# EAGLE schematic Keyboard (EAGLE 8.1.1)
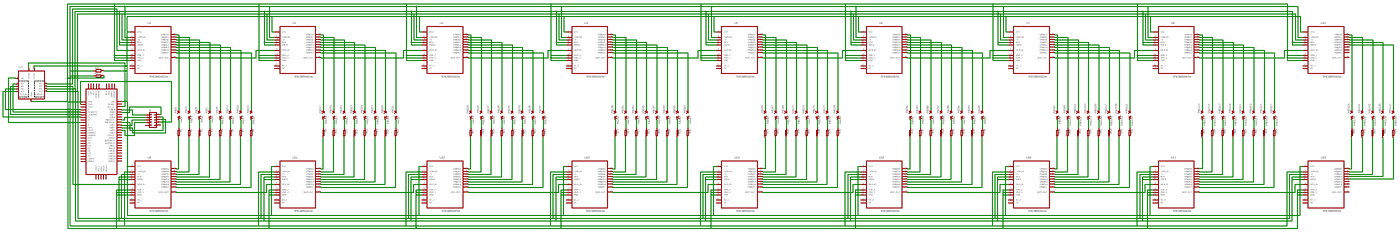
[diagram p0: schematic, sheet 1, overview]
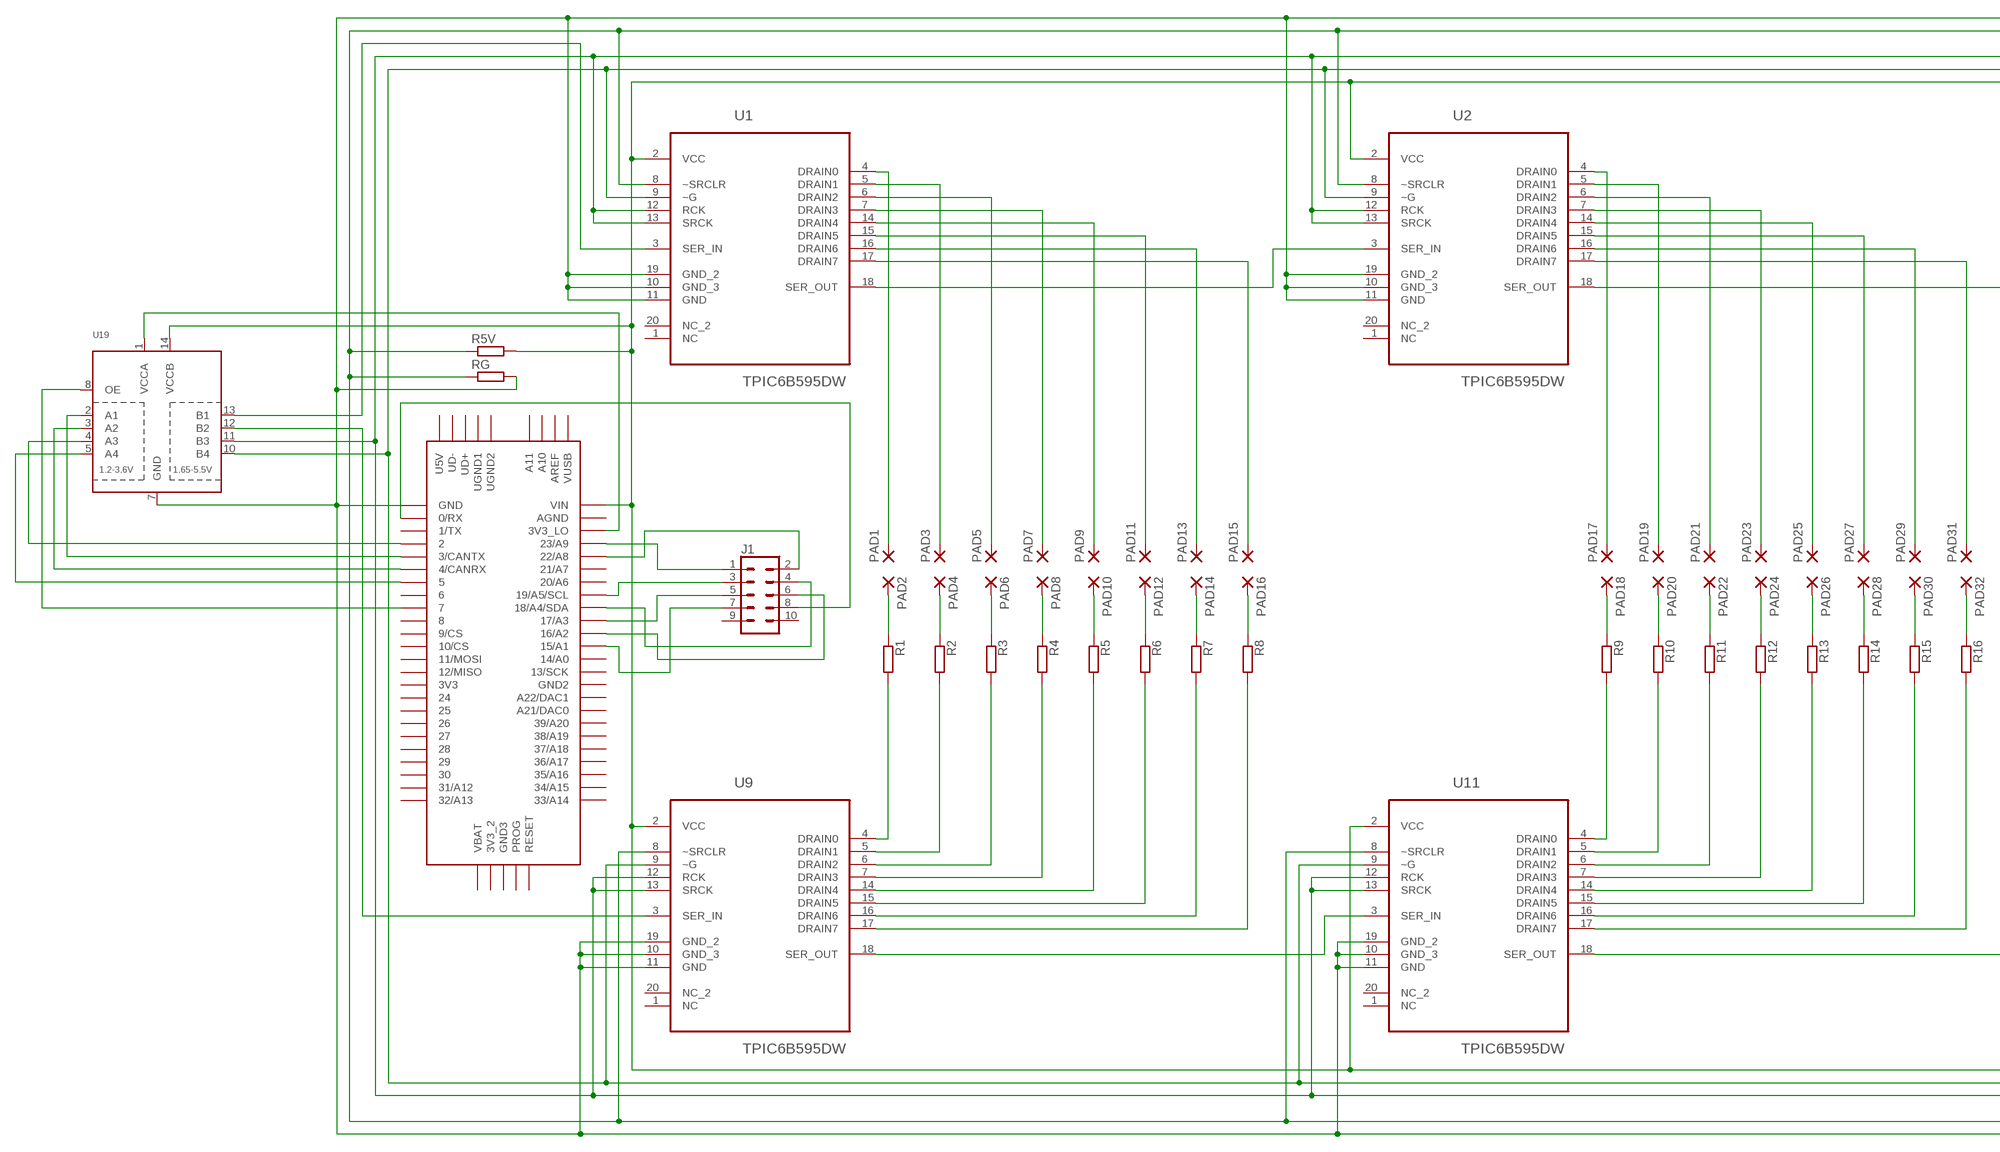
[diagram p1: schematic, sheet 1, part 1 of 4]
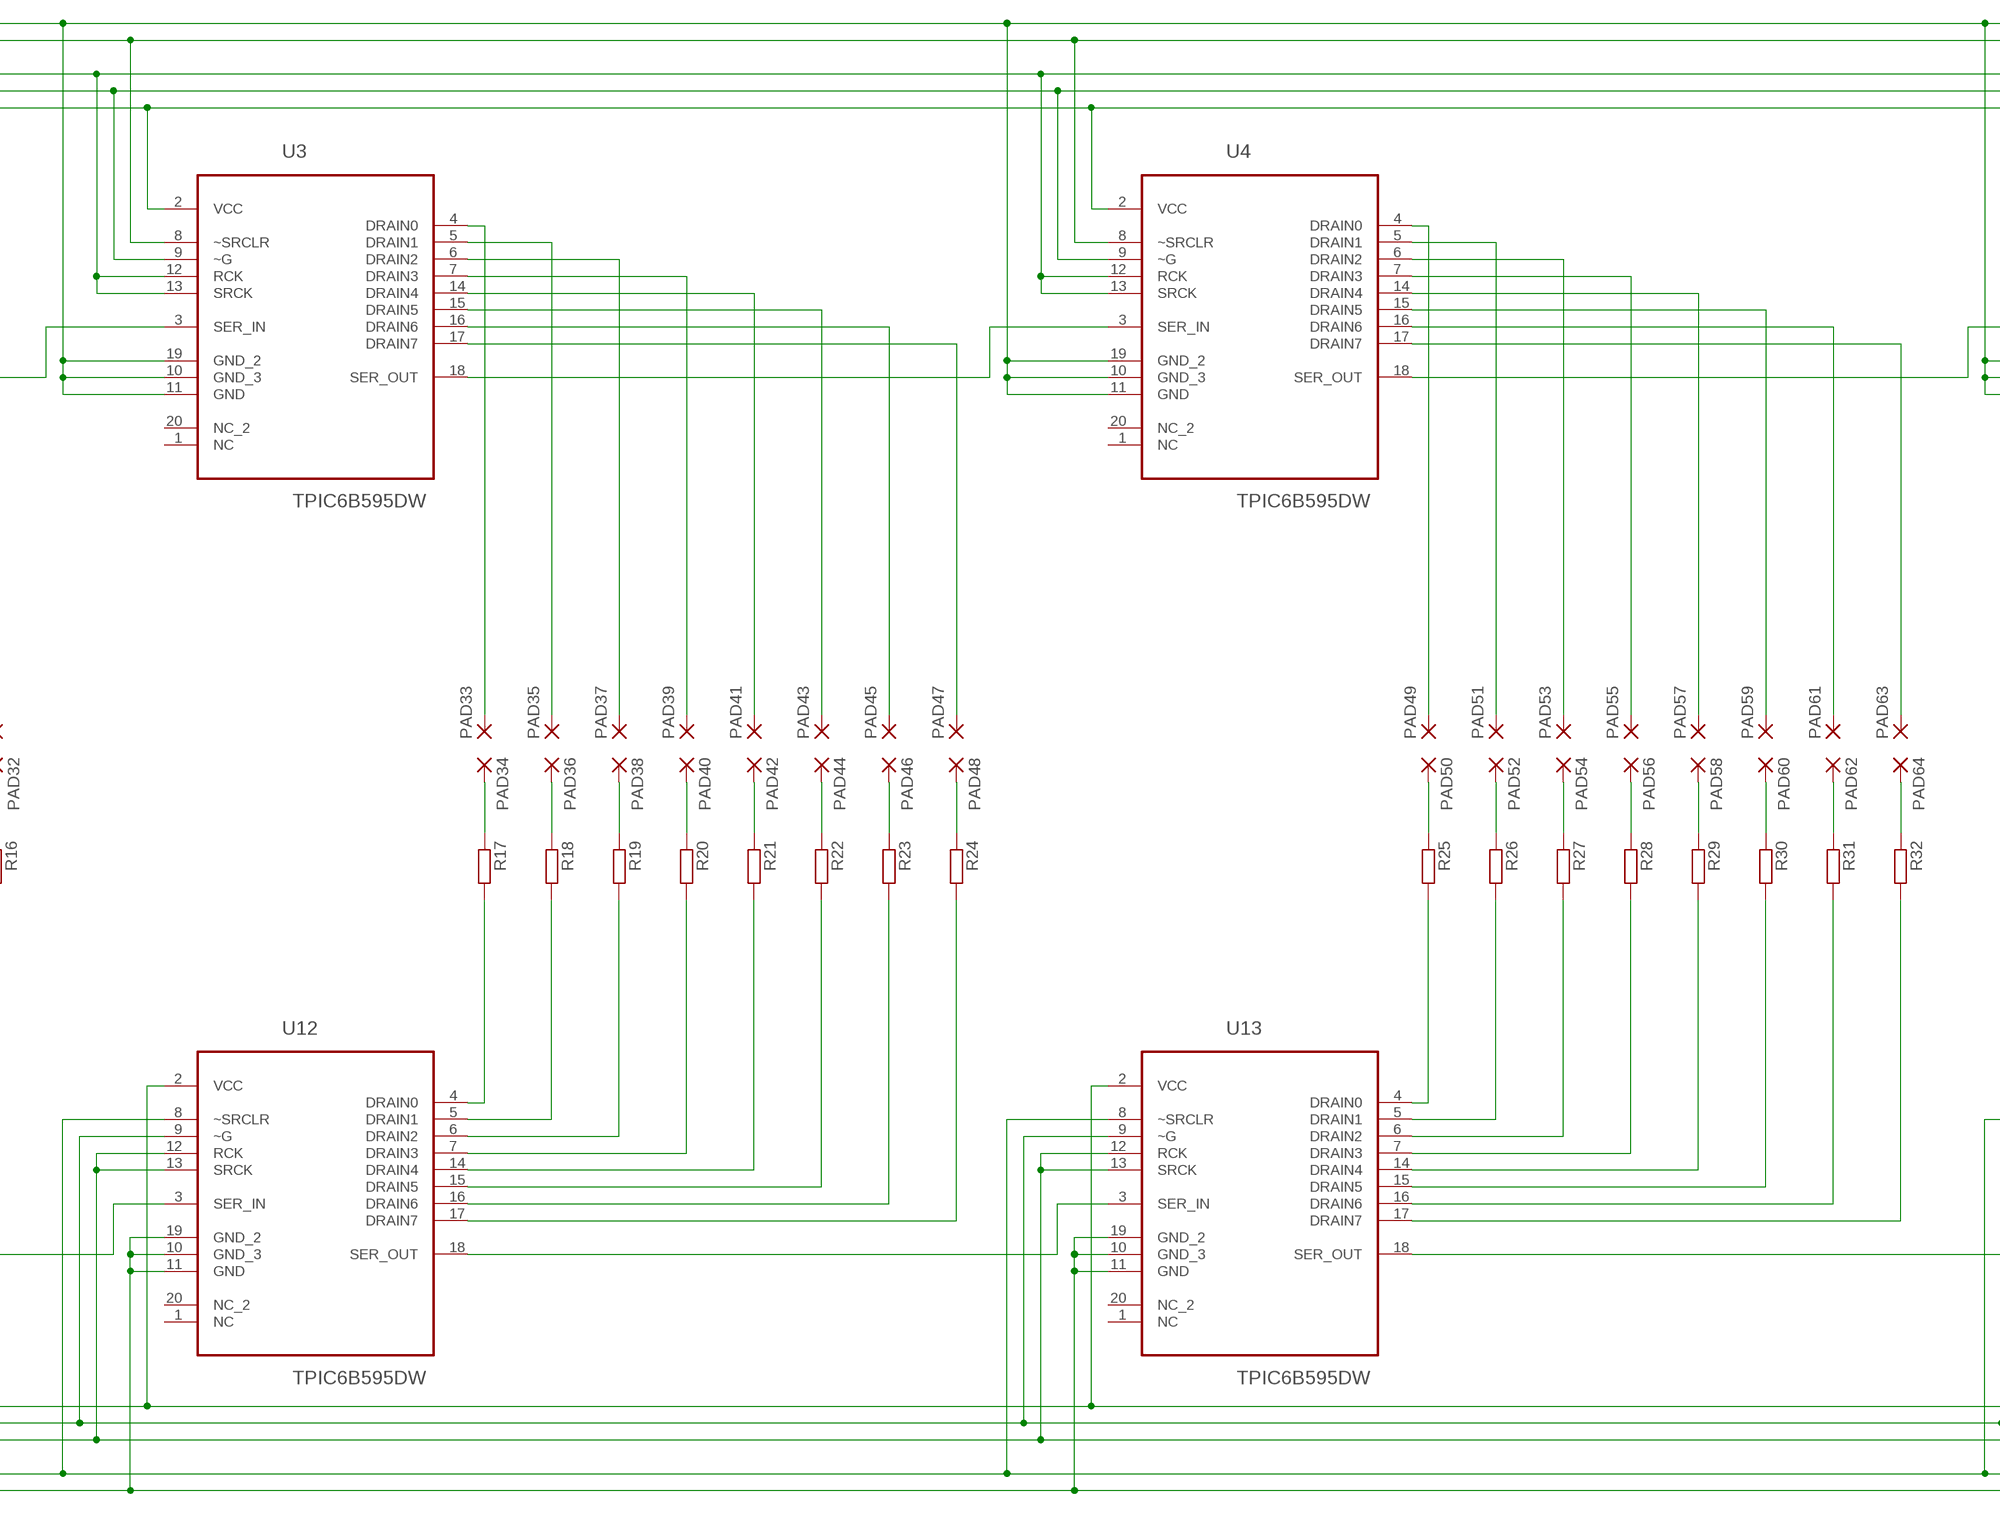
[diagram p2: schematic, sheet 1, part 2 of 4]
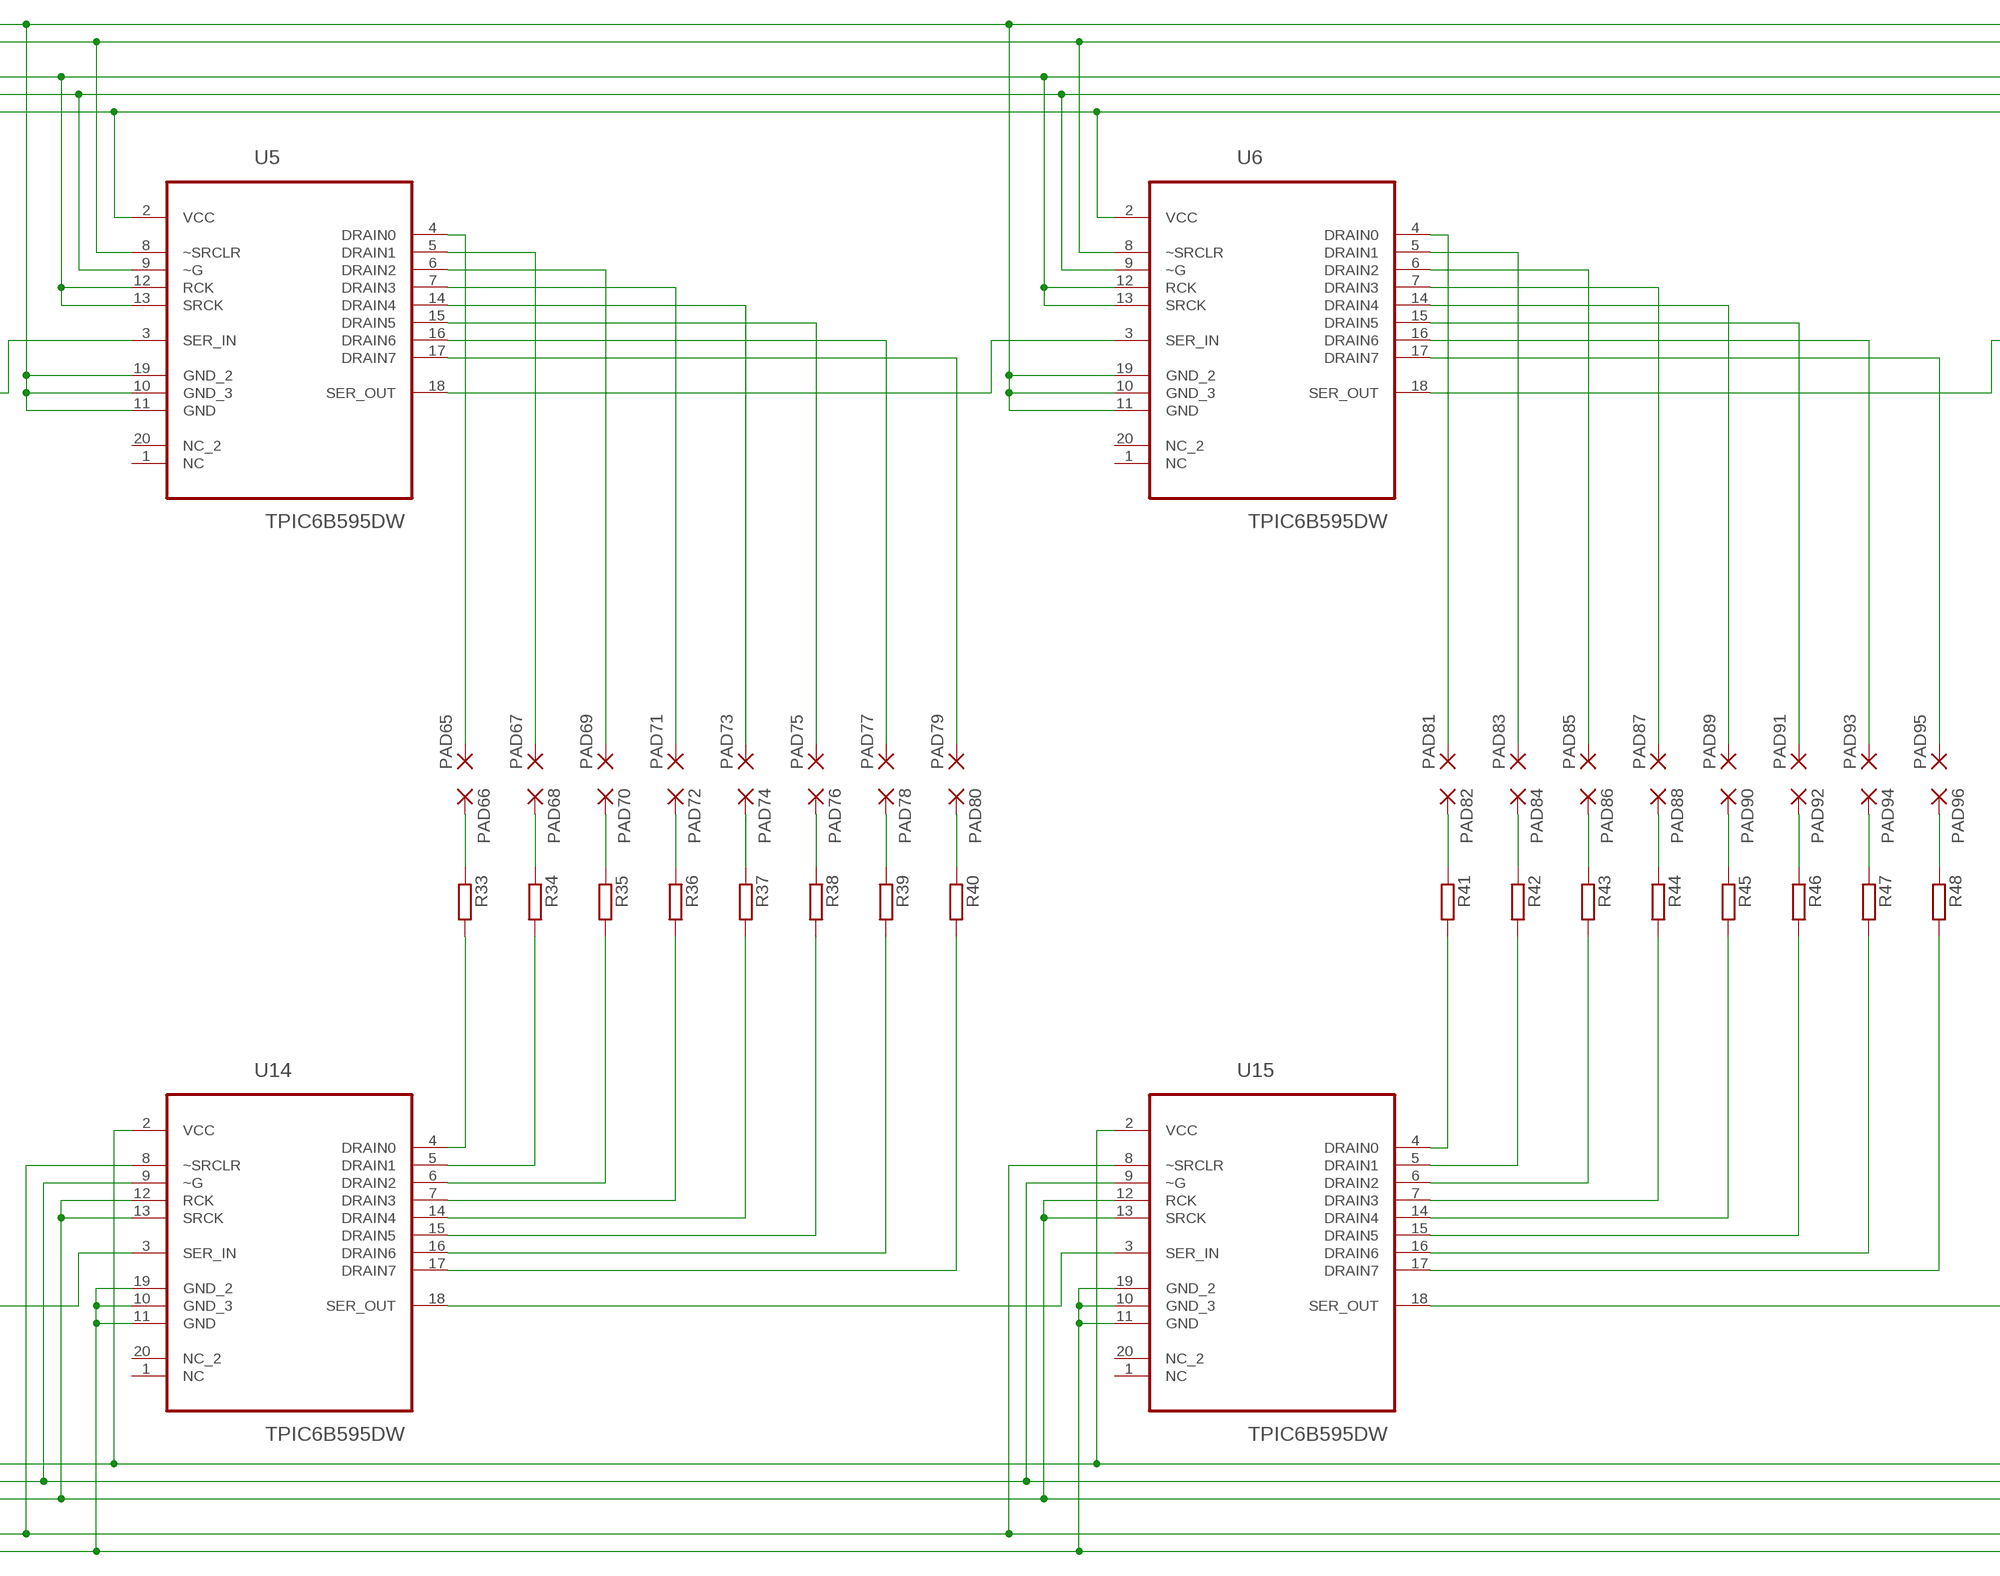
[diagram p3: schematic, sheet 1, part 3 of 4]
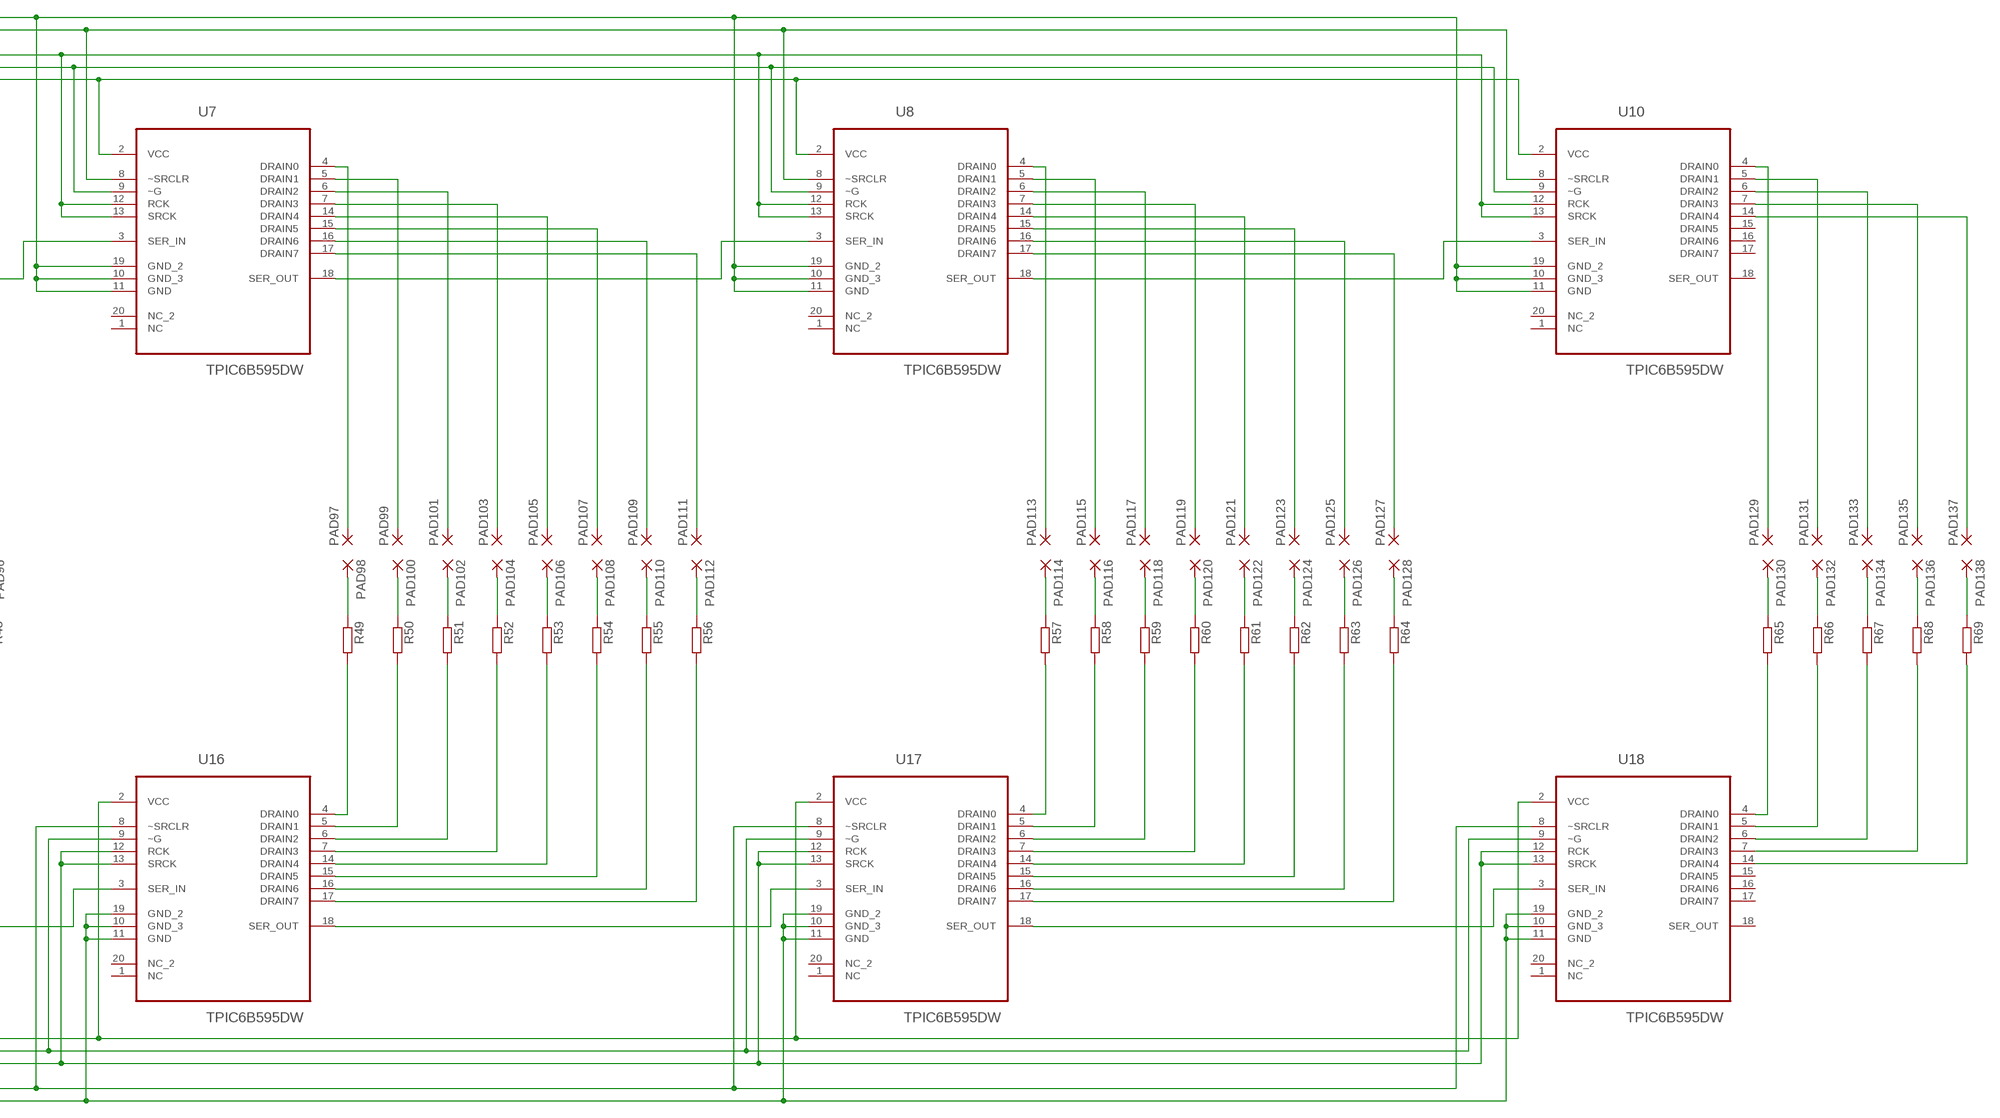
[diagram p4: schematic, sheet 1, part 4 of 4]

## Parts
J1  CONN_05X2SHD  [2X5-SHROUDED]
PAD1  1,6/0,8  [1,6/0,8]
PAD2  1,6/0,8  [1,6/0,8]
PAD3  1,6/0,8  [1,6/0,8]
PAD4  1,6/0,8  [1,6/0,8]
PAD5  1,6/0,8  [1,6/0,8]
PAD6  1,6/0,8  [1,6/0,8]
PAD7  1,6/0,8  [1,6/0,8]
PAD8  1,6/0,8  [1,6/0,8]
PAD9  1,6/0,8  [1,6/0,8]
PAD10  1,6/0,8  [1,6/0,8]
PAD11  1,6/0,8  [1,6/0,8]
PAD12  1,6/0,8  [1,6/0,8]
PAD13  1,6/0,8  [1,6/0,8]
PAD14  1,6/0,8  [1,6/0,8]
PAD15  1,6/0,8  [1,6/0,8]
PAD16  1,6/0,8  [1,6/0,8]
PAD17  1,6/0,8  [1,6/0,8]
PAD18  1,6/0,8  [1,6/0,8]
PAD19  1,6/0,8  [1,6/0,8]
PAD20  1,6/0,8  [1,6/0,8]
PAD21  1,6/0,8  [1,6/0,8]
PAD22  1,6/0,8  [1,6/0,8]
PAD23  1,6/0,8  [1,6/0,8]
PAD24  1,6/0,8  [1,6/0,8]
PAD25  1,6/0,8  [1,6/0,8]
PAD26  1,6/0,8  [1,6/0,8]
PAD27  1,6/0,8  [1,6/0,8]
PAD28  1,6/0,8  [1,6/0,8]
PAD29  1,6/0,8  [1,6/0,8]
PAD30  1,6/0,8  [1,6/0,8]
PAD31  1,6/0,8  [1,6/0,8]
PAD32  1,6/0,8  [1,6/0,8]
PAD33  1,6/0,8  [1,6/0,8]
PAD34  1,6/0,8  [1,6/0,8]
PAD35  1,6/0,8  [1,6/0,8]
PAD36  1,6/0,8  [1,6/0,8]
PAD37  1,6/0,8  [1,6/0,8]
PAD38  1,6/0,8  [1,6/0,8]
PAD39  1,6/0,8  [1,6/0,8]
PAD40  1,6/0,8  [1,6/0,8]
PAD41  1,6/0,8  [1,6/0,8]
PAD42  1,6/0,8  [1,6/0,8]
PAD43  1,6/0,8  [1,6/0,8]
PAD44  1,6/0,8  [1,6/0,8]
PAD45  1,6/0,8  [1,6/0,8]
PAD46  1,6/0,8  [1,6/0,8]
PAD47  1,6/0,8  [1,6/0,8]
PAD48  1,6/0,8  [1,6/0,8]
PAD49  1,6/0,8  [1,6/0,8]
PAD50  1,6/0,8  [1,6/0,8]
PAD51  1,6/0,8  [1,6/0,8]
PAD52  1,6/0,8  [1,6/0,8]
PAD53  1,6/0,8  [1,6/0,8]
PAD54  1,6/0,8  [1,6/0,8]
PAD55  1,6/0,8  [1,6/0,8]
PAD56  1,6/0,8  [1,6/0,8]
PAD57  1,6/0,8  [1,6/0,8]
PAD58  1,6/0,8  [1,6/0,8]
PAD59  1,6/0,8  [1,6/0,8]
PAD60  1,6/0,8  [1,6/0,8]
PAD61  1,6/0,8  [1,6/0,8]
PAD62  1,6/0,8  [1,6/0,8]
PAD63  1,6/0,8  [1,6/0,8]
PAD64  1,6/0,8  [1,6/0,8]
PAD65  1,6/0,8  [1,6/0,8]
PAD66  1,6/0,8  [1,6/0,8]
PAD67  1,6/0,8  [1,6/0,8]
PAD68  1,6/0,8  [1,6/0,8]
PAD69  1,6/0,8  [1,6/0,8]
PAD70  1,6/0,8  [1,6/0,8]
PAD71  1,6/0,8  [1,6/0,8]
PAD72  1,6/0,8  [1,6/0,8]
PAD73  1,6/0,8  [1,6/0,8]
PAD74  1,6/0,8  [1,6/0,8]
PAD75  1,6/0,8  [1,6/0,8]
PAD76  1,6/0,8  [1,6/0,8]
PAD77  1,6/0,8  [1,6/0,8]
PAD78  1,6/0,8  [1,6/0,8]
PAD79  1,6/0,8  [1,6/0,8]
PAD80  1,6/0,8  [1,6/0,8]
PAD81  1,6/0,8  [1,6/0,8]
PAD82  1,6/0,8  [1,6/0,8]
PAD83  1,6/0,8  [1,6/0,8]
PAD84  1,6/0,8  [1,6/0,8]
PAD85  1,6/0,8  [1,6/0,8]
PAD86  1,6/0,8  [1,6/0,8]
PAD87  1,6/0,8  [1,6/0,8]
PAD88  1,6/0,8  [1,6/0,8]
PAD89  1,6/0,8  [1,6/0,8]
PAD90  1,6/0,8  [1,6/0,8]
PAD91  1,6/0,8  [1,6/0,8]
PAD92  1,6/0,8  [1,6/0,8]
PAD93  1,6/0,8  [1,6/0,8]
PAD94  1,6/0,8  [1,6/0,8]
PAD95  1,6/0,8  [1,6/0,8]
PAD96  1,6/0,8  [1,6/0,8]
PAD97  1,6/0,8  [1,6/0,8]
PAD98  1,6/0,8  [1,6/0,8]
PAD99  1,6/0,8  [1,6/0,8]
PAD100  1,6/0,8  [1,6/0,8]
PAD101  1,6/0,8  [1,6/0,8]
PAD102  1,6/0,8  [1,6/0,8]
PAD103  1,6/0,8  [1,6/0,8]
PAD104  1,6/0,8  [1,6/0,8]
PAD105  1,6/0,8  [1,6/0,8]
PAD106  1,6/0,8  [1,6/0,8]
PAD107  1,6/0,8  [1,6/0,8]
PAD108  1,6/0,8  [1,6/0,8]
PAD109  1,6/0,8  [1,6/0,8]
PAD110  1,6/0,8  [1,6/0,8]
PAD111  1,6/0,8  [1,6/0,8]
PAD112  1,6/0,8  [1,6/0,8]
PAD113  1,6/0,8  [1,6/0,8]
PAD114  1,6/0,8  [1,6/0,8]
PAD115  1,6/0,8  [1,6/0,8]
PAD116  1,6/0,8  [1,6/0,8]
PAD117  1,6/0,8  [1,6/0,8]
PAD118  1,6/0,8  [1,6/0,8]
PAD119  1,6/0,8  [1,6/0,8]
PAD120  1,6/0,8  [1,6/0,8]
PAD121  1,6/0,8  [1,6/0,8]
PAD122  1,6/0,8  [1,6/0,8]
PAD123  1,6/0,8  [1,6/0,8]
PAD124  1,6/0,8  [1,6/0,8]
PAD125  1,6/0,8  [1,6/0,8]
PAD126  1,6/0,8  [1,6/0,8]
PAD127  1,6/0,8  [1,6/0,8]
PAD128  1,6/0,8  [1,6/0,8]
PAD129  1,6/0,8  [1,6/0,8]
PAD130  1,6/0,8  [1,6/0,8]
PAD131  1,6/0,8  [1,6/0,8]
PAD132  1,6/0,8  [1,6/0,8]
PAD133  1,6/0,8  [1,6/0,8]
PAD134  1,6/0,8  [1,6/0,8]
PAD135  1,6/0,8  [1,6/0,8]
PAD136  1,6/0,8  [1,6/0,8]
PAD137  1,6/0,8  [1,6/0,8]
PAD138  1,6/0,8  [1,6/0,8]
R1  R  [R0805]
R2  R  [R0805]
R3  R  [R0805]
R4  R  [R0805]
R5  R  [R0805]
R5V  R  [R0805]
R6  R  [R0805]
R7  R  [R0805]
R8  R  [R0805]
R9  R  [R0805]
R10  R  [R0805]
R11  R  [R0805]
R12  R  [R0805]
R13  R  [R0805]
R14  R  [R0805]
R15  R  [R0805]
R16  R  [R0805]
R17  R  [R0805]
R18  R  [R0805]
R19  R  [R0805]
R20  R  [R0805]
R21  R  [R0805]
R22  R  [R0805]
R23  R  [R0805]
R24  R  [R0805]
R25  R  [R0805]
R26  R  [R0805]
R27  R  [R0805]
R28  R  [R0805]
R29  R  [R0805]
R30  R  [R0805]
R31  R  [R0805]
R32  R  [R0805]
R33  R  [R0805]
R34  R  [R0805]
R35  R  [R0805]
R36  R  [R0805]
R37  R  [R0805]
R38  R  [R0805]
R39  R  [R0805]
R40  R  [R0805]
R41  R  [R0805]
R42  R  [R0805]
R43  R  [R0805]
R44  R  [R0805]
R45  R  [R0805]
R46  R  [R0805]
R47  R  [R0805]
R48  R  [R0805]
R49  R  [R0805]
R50  R  [R0805]
R51  R  [R0805]
R52  R  [R0805]
R53  R  [R0805]
R54  R  [R0805]
R55  R  [R0805]
R56  R  [R0805]
R57  R  [R0805]
R58  R  [R0805]
R59  R  [R0805]
R60  R  [R0805]
R61  R  [R0805]
R62  R  [R0805]
R63  R  [R0805]
R64  R  [R0805]
R65  R  [R0805]
R66  R  [R0805]
R67  R  [R0805]
R68  R  [R0805]
R69  R  [R0805]
RG  R  [R0805]
U1  TPIC6B595DW  [SOIC127P1030X265-20N]
U2  TPIC6B595DW  [SOIC127P1030X265-20N]
U3  TPIC6B595DW  [SOIC127P1030X265-20N]
U4  TPIC6B595DW  [SOIC127P1030X265-20N]
U5  TPIC6B595DW  [SOIC127P1030X265-20N]
U6  TPIC6B595DW  [SOIC127P1030X265-20N]
U7  TPIC6B595DW  [SOIC127P1030X265-20N]
U8  TPIC6B595DW  [SOIC127P1030X265-20N]
U9  TPIC6B595DW  [SOIC127P1030X265-20N]
U10  TPIC6B595DW  [SOIC127P1030X265-20N]
U11  TPIC6B595DW  [SOIC127P1030X265-20N]
U12  TPIC6B595DW  [SOIC127P1030X265-20N]
U13  TPIC6B595DW  [SOIC127P1030X265-20N]
U14  TPIC6B595DW  [SOIC127P1030X265-20N]
U15  TPIC6B595DW  [SOIC127P1030X265-20N]
U16  TPIC6B595DW  [SOIC127P1030X265-20N]
U17  TPIC6B595DW  [SOIC127P1030X265-20N]
U18  TPIC6B595DW  [SOIC127P1030X265-20N]
U19  TXB0104PWRSOIC14  [SO14]
U$59  TEENSY_3.5/3.6  [TEENSY_3.5/3.6]

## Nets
N$1: PAD2.1(P) R1.1
N$2: U1.18(SER_OUT) U2.3(SER_IN)
N$3: U1.12(RCK) U1.13(SRCK) U2.12(RCK) U2.13(SRCK) U3.12(RCK) U3.13(SRCK) U4.12(RCK) U4.13(SRCK) U5.12(RCK) U5.13(SRCK) U6.12(RCK) U6.13(SRCK) U7.12(RCK) U7.13(SRCK) U8.12(RCK) U8.13(SRCK) U9.12(RCK) U9.13(SRCK) U10.12(RCK) U10.13(SRCK) U11.12(RCK) U11.13(SRCK) U12.12(RCK) U12.13(SRCK) U13.12(RCK) U13.13(SRCK) U14.12(RCK) U14.13(SRCK) U15.12(RCK) U15.13(SRCK) U16.12(RCK) U16.13(SRCK) U17.12(RCK) U17.13(SRCK) U18.12(RCK) U18.13(SRCK) U19.11(B3)
N$4: PAD4.1(P) R2.1
N$5: PAD6.1(P) R3.1
N$6: PAD8.1(P) R4.1
N$7: PAD10.1(P) R5.1
N$8: PAD12.1(P) R6.1
N$9: PAD14.1(P) R7.1
N$10: PAD16.1(P) R8.1
N$11: PAD18.1(P) R9.1
N$12: U1.9(~G) U2.9(~G) U3.9(~G) U4.9(~G) U5.9(~G) U6.9(~G) U7.9(~G) U8.9(~G) U9.9(~G) U10.9(~G) U11.9(~G) U12.9(~G) U13.9(~G) U14.9(~G) U15.9(~G) U16.9(~G) U17.9(~G) U18.9(~G) U19.10(B4)
N$13: PAD20.1(P) R10.1
N$14: PAD22.1(P) R11.1
N$15: PAD24.1(P) R12.1
N$16: PAD26.1(P) R13.1
N$17: PAD28.1(P) R14.1
N$18: PAD30.1(P) R15.1
N$19: PAD32.1(P) R16.1
N$20: PAD34.1(P) R17.1
N$21: PAD36.1(P) R18.1
N$22: PAD38.1(P) R19.1
N$23: PAD40.1(P) R20.1
N$24: PAD42.1(P) R21.1
N$25: PAD44.1(P) R22.1
N$26: PAD46.1(P) R23.1
N$27: PAD48.1(P) R24.1
N$28: PAD50.1(P) R25.1
N$29: PAD52.1(P) R26.1
N$30: PAD54.1(P) R27.1
N$31: PAD56.1(P) R28.1
N$32: PAD58.1(P) R29.1
N$33: PAD60.1(P) R30.1
N$34: PAD62.1(P) R31.1
N$35: PAD64.1(P) R32.1
N$36: PAD66.1(P) R33.1
N$37: PAD68.1(P) R34.1
N$38: PAD70.1(P) R35.1
N$39: PAD72.1(P) R36.1
N$40: PAD74.1(P) R37.1
N$41: PAD76.1(P) R38.1
N$42: PAD78.1(P) R39.1
N$43: PAD80.1(P) R40.1
N$44: PAD82.1(P) R41.1
N$45: PAD84.1(P) R42.1
N$46: PAD86.1(P) R43.1
N$47: PAD88.1(P) R44.1
N$48: PAD90.1(P) R45.1
N$49: PAD92.1(P) R46.1
N$50: PAD94.1(P) R47.1
N$51: PAD96.1(P) R48.1
N$52: PAD98.1(P) R49.1
N$53: PAD100.1(P) R50.1
N$54: PAD102.1(P) R51.1
N$55: PAD104.1(P) R52.1
N$56: PAD106.1(P) R53.1
N$57: PAD108.1(P) R54.1
N$58: PAD110.1(P) R55.1
N$59: PAD112.1(P) R56.1
N$60: PAD114.1(P) R57.1
N$61: R5V.2 U1.2(VCC) U2.2(VCC) U3.2(VCC) U4.2(VCC) U5.2(VCC) U6.2(VCC) U7.2(VCC) U8.2(VCC) U9.2(VCC) U10.2(VCC) U11.2(VCC) U12.2(VCC) U13.2(VCC) U14.2(VCC) U15.2(VCC) U16.2(VCC) U17.2(VCC) U18.2(VCC) U19.14(VCCB) U$59.VIN
N$62: U19.4(A3) U$59.2
N$63: R5V.1 RG.1 U1.8(~SRCLR) U2.8(~SRCLR) U3.8(~SRCLR) U4.8(~SRCLR) U5.8(~SRCLR) U6.8(~SRCLR) U7.8(~SRCLR) U8.8(~SRCLR) U9.8(~SRCLR) U10.8(~SRCLR) U11.8(~SRCLR) U12.8(~SRCLR) U13.8(~SRCLR) U14.8(~SRCLR) U15.8(~SRCLR) U16.8(~SRCLR) U17.8(~SRCLR) U18.8(~SRCLR)
N$64: U1.3(SER_IN) U19.13(B1)
N$65: U2.18(SER_OUT) U3.3(SER_IN)
N$66: R68.2 U18.7(DRAIN3)
N$67: R69.2 U18.14(DRAIN4)
N$68: PAD129.1(P) U10.4(DRAIN0)
N$69: PAD131.1(P) U10.5(DRAIN1)
N$70: U3.18(SER_OUT) U4.3(SER_IN)
N$71: U4.18(SER_OUT) U5.3(SER_IN)
N$72: U5.18(SER_OUT) U6.3(SER_IN)
N$73: U6.18(SER_OUT) U7.3(SER_IN)
N$74: U7.18(SER_OUT) U8.3(SER_IN)
N$75: U8.18(SER_OUT) U10.3(SER_IN)
N$76: U19.1(VCCA) U$59.3V3_LO
N$77: U19.2(A1) U$59.3/CANTX
N$78: U9.3(SER_IN) U19.12(B2)
N$79: U19.8(OE) U$59.7
N$80: PAD116.1(P) R58.1
N$81: PAD118.1(P) R59.1
N$82: PAD120.1(P) R60.1
N$83: PAD122.1(P) R61.1
N$84: PAD124.1(P) R62.1
N$85: PAD126.1(P) R63.1
N$86: PAD128.1(P) R64.1
N$87: U9.18(SER_OUT) U11.3(SER_IN)
N$88: U11.18(SER_OUT) U12.3(SER_IN)
N$89: U12.18(SER_OUT) U13.3(SER_IN)
N$90: U13.18(SER_OUT) U14.3(SER_IN)
N$91: U14.18(SER_OUT) U15.3(SER_IN)
N$92: U15.18(SER_OUT) U16.3(SER_IN)
N$93: U16.18(SER_OUT) U17.3(SER_IN)
N$94: U17.18(SER_OUT) U18.3(SER_IN)
N$95: RG.2 U1.10(GND_3) U1.11(GND) U1.19(GND_2) U2.10(GND_3) U2.11(GND) U2.19(GND_2) U3.10(GND_3) U3.11(GND) U3.19(GND_2) U4.10(GND_3) U4.11(GND) U4.19(GND_2) U5.10(GND_3) U5.11(GND) U5.19(GND_2) U6.10(GND_3) U6.11(GND) U6.19(GND_2) U7.10(GND_3) U7.11(GND) U7.19(GND_2) U8.10(GND_3) U8.11(GND) U8.19(GND_2) U9.10(GND_3) U9.11(GND) U9.19(GND_2) U10.10(GND_3) U10.11(GND) U10.19(GND_2) U11.10(GND_3) U11.11(GND) U11.19(GND_2) U12.10(GND_3) U12.11(GND) U12.19(GND_2) U13.10(GND_3) U13.11(GND) U13.19(GND_2) U14.10(GND_3) U14.11(GND) U14.19(GND_2) U15.10(GND_3) U15.11(GND) U15.19(GND_2) U16.10(GND_3) U16.11(GND) U16.19(GND_2) U17.10(GND_3) U17.11(GND) U17.19(GND_2) U18.10(GND_3) U18.11(GND) U18.19(GND_2) U19.7(GND) U$59.GND
N$96: U19.5(A4) U$59.5
N$97: PAD130.1(P) R65.1
N$98: PAD1.1(P) U1.4(DRAIN0)
N$99: PAD3.1(P) U1.5(DRAIN1)
N$100: PAD5.1(P) U1.6(DRAIN2)
N$101: PAD7.1(P) U1.7(DRAIN3)
N$102: PAD9.1(P) U1.14(DRAIN4)
N$103: PAD11.1(P) U1.15(DRAIN5)
N$104: PAD13.1(P) U1.16(DRAIN6)
N$105: PAD15.1(P) U1.17(DRAIN7)
N$106: R1.2 U9.4(DRAIN0)
N$107: R2.2 U9.5(DRAIN1)
N$108: R3.2 U9.6(DRAIN2)
N$109: R4.2 U9.7(DRAIN3)
N$110: R5.2 U9.14(DRAIN4)
N$111: R6.2 U9.15(DRAIN5)
N$112: R7.2 U9.16(DRAIN6)
N$113: R8.2 U9.17(DRAIN7)
N$114: R9.2 U11.4(DRAIN0)
N$115: R10.2 U11.5(DRAIN1)
N$116: R11.2 U11.6(DRAIN2)
N$117: R12.2 U11.7(DRAIN3)
N$118: R13.2 U11.14(DRAIN4)
N$119: R14.2 U11.15(DRAIN5)
N$120: R15.2 U11.16(DRAIN6)
N$121: R16.2 U11.17(DRAIN7)
N$122: PAD17.1(P) U2.4(DRAIN0)
N$123: PAD19.1(P) U2.5(DRAIN1)
N$124: PAD21.1(P) U2.6(DRAIN2)
N$125: PAD23.1(P) U2.7(DRAIN3)
N$126: PAD25.1(P) U2.14(DRAIN4)
N$127: PAD27.1(P) U2.15(DRAIN5)
N$128: PAD29.1(P) U2.16(DRAIN6)
N$129: PAD31.1(P) U2.17(DRAIN7)
N$130: PAD33.1(P) U3.4(DRAIN0)
N$131: PAD35.1(P) U3.5(DRAIN1)
N$132: PAD37.1(P) U3.6(DRAIN2)
N$133: PAD39.1(P) U3.7(DRAIN3)
N$134: PAD41.1(P) U3.14(DRAIN4)
N$135: PAD43.1(P) U3.15(DRAIN5)
N$136: PAD45.1(P) U3.16(DRAIN6)
N$137: PAD47.1(P) U3.17(DRAIN7)
N$138: R17.2 U12.4(DRAIN0)
N$139: R18.2 U12.5(DRAIN1)
N$140: R19.2 U12.6(DRAIN2)
N$141: R20.2 U12.7(DRAIN3)
N$142: R21.2 U12.14(DRAIN4)
N$143: R22.2 U12.15(DRAIN5)
N$144: R23.2 U12.16(DRAIN6)
N$145: R24.2 U12.17(DRAIN7)
N$146: R25.2 U13.4(DRAIN0)
N$147: R26.2 U13.5(DRAIN1)
N$148: R27.2 U13.6(DRAIN2)
N$149: U19.3(A2) U$59.4/CANRX
N$150: R28.2 U13.7(DRAIN3)
N$151: R29.2 U13.14(DRAIN4)
N$152: R30.2 U13.15(DRAIN5)
N$153: R31.2 U13.16(DRAIN6)
N$154: R32.2 U13.17(DRAIN7)
N$155: PAD49.1(P) U4.4(DRAIN0)
N$156: PAD51.1(P) U4.5(DRAIN1)
N$157: PAD53.1(P) U4.6(DRAIN2)
N$158: PAD55.1(P) U4.7(DRAIN3)
N$159: PAD57.1(P) U4.14(DRAIN4)
N$160: PAD59.1(P) U4.15(DRAIN5)
N$161: PAD61.1(P) U4.16(DRAIN6)
N$162: PAD63.1(P) U4.17(DRAIN7)
N$163: PAD65.1(P) U5.4(DRAIN0)
N$164: PAD67.1(P) U5.5(DRAIN1)
N$165: PAD69.1(P) U5.6(DRAIN2)
N$166: PAD71.1(P) U5.7(DRAIN3)
N$167: PAD73.1(P) U5.14(DRAIN4)
N$168: PAD75.1(P) U5.15(DRAIN5)
N$169: PAD77.1(P) U5.16(DRAIN6)
N$170: PAD79.1(P) U5.17(DRAIN7)
N$171: R33.2 U14.4(DRAIN0)
N$172: R34.2 U14.5(DRAIN1)
N$173: R35.2 U14.6(DRAIN2)
N$174: R36.2 U14.7(DRAIN3)
N$175: R37.2 U14.14(DRAIN4)
N$176: R38.2 U14.15(DRAIN5)
N$177: R39.2 U14.16(DRAIN6)
N$178: R40.2 U14.17(DRAIN7)
N$179: R41.2 U15.4(DRAIN0)
N$180: R42.2 U15.5(DRAIN1)
N$181: R43.2 U15.6(DRAIN2)
N$182: R44.2 U15.7(DRAIN3)
N$183: R45.2 U15.14(DRAIN4)
N$184: R46.2 U15.15(DRAIN5)
N$185: R47.2 U15.16(DRAIN6)
N$186: R48.2 U15.17(DRAIN7)
N$187: PAD81.1(P) U6.4(DRAIN0)
N$188: PAD83.1(P) U6.5(DRAIN1)
N$189: PAD85.1(P) U6.6(DRAIN2)
N$190: PAD87.1(P) U6.7(DRAIN3)
N$191: PAD89.1(P) U6.14(DRAIN4)
N$192: PAD91.1(P) U6.15(DRAIN5)
N$193: PAD93.1(P) U6.16(DRAIN6)
N$194: PAD95.1(P) U6.17(DRAIN7)
N$195: R49.2 U16.4(DRAIN0)
N$196: R50.2 U16.5(DRAIN1)
N$197: R51.2 U16.6(DRAIN2)
N$198: R52.2 U16.7(DRAIN3)
N$199: R53.2 U16.14(DRAIN4)
N$200: R54.2 U16.15(DRAIN5)
N$201: R55.2 U16.16(DRAIN6)
N$202: R56.2 U16.17(DRAIN7)
N$203: PAD97.1(P) U7.4(DRAIN0)
N$204: PAD99.1(P) U7.5(DRAIN1)
N$205: PAD101.1(P) U7.6(DRAIN2)
N$206: PAD103.1(P) U7.7(DRAIN3)
N$207: PAD105.1(P) U7.14(DRAIN4)
N$208: PAD107.1(P) U7.15(DRAIN5)
N$209: PAD109.1(P) U7.16(DRAIN6)
N$210: PAD111.1(P) U7.17(DRAIN7)
N$211: PAD113.1(P) U8.4(DRAIN0)
N$212: PAD115.1(P) U8.5(DRAIN1)
N$213: PAD117.1(P) U8.6(DRAIN2)
N$214: PAD119.1(P) U8.7(DRAIN3)
N$215: PAD121.1(P) U8.14(DRAIN4)
N$216: PAD123.1(P) U8.15(DRAIN5)
N$217: PAD125.1(P) U8.16(DRAIN6)
N$218: PAD127.1(P) U8.17(DRAIN7)
N$219: R57.2 U17.4(DRAIN0)
N$220: R58.2 U17.5(DRAIN1)
N$221: R59.2 U17.6(DRAIN2)
N$222: R60.2 U17.7(DRAIN3)
N$223: R61.2 U17.14(DRAIN4)
N$224: R62.2 U17.15(DRAIN5)
N$225: R63.2 U17.16(DRAIN6)
N$226: R64.2 U17.17(DRAIN7)
N$227: R65.2 U18.4(DRAIN0)
N$228: R66.2 U18.5(DRAIN1)
N$229: R67.2 U18.6(DRAIN2)
N$230: PAD132.1(P) R66.1
N$231: PAD134.1(P) R67.1
N$232: PAD136.1(P) R68.1
N$233: PAD138.1(P) R69.1
N$234: PAD133.1(P) U10.6(DRAIN2)
N$235: PAD135.1(P) U10.7(DRAIN3)
N$236: PAD137.1(P) U10.14(DRAIN4)
N$237: J1.1 U$59.23/A9
N$238: J1.2 U$59.22/A8
N$239: J1.3 U$59.19/A5/SCL
N$240: J1.4 U$59.18/A4/SDA
N$241: J1.5 U$59.17/A3
N$242: J1.6 U$59.16/A2
N$243: J1.7 U$59.15/A1
N$244: J1.8 U$59.0/RX
Unconnected: J1.9 J1.10 U1.1(NC) U1.20(NC_2) U2.1(NC) U2.20(NC_2) U3.1(NC) U3.20(NC_2) U4.1(NC) U4.20(NC_2) U5.1(NC) U5.20(NC_2) U6.1(NC) U6.20(NC_2) U7.1(NC) U7.20(NC_2) U8.1(NC) U8.20(NC_2) U9.1(NC) U9.20(NC_2) U10.1(NC) U10.15(DRAIN5) U10.16(DRAIN6) U10.17(DRAIN7) U10.18(SER_OUT) U10.20(NC_2) U11.1(NC) U11.20(NC_2) U12.1(NC) U12.20(NC_2) U13.1(NC) U13.20(NC_2) U14.1(NC) U14.20(NC_2) U15.1(NC) U15.20(NC_2) U16.1(NC) U16.20(NC_2) U17.1(NC) U17.20(NC_2) U18.1(NC) U18.15(DRAIN5) U18.16(DRAIN6) U18.17(DRAIN7) U18.18(SER_OUT) U18.20(NC_2) U$59.1/TX U$59.3V3 U$59.3V3_2 U$59.6 U$59.8 U$59.9/CS U$59.10/CS U$59.11/MOSI U$59.12/MISO U$59.13/SCK U$59.14/A0 U$59.20/A6 U$59.21/A7 U$59.21/DAC0(A21/DAC0) U$59.24 U$59.25 U$59.26 U$59.27 U$59.28 U$59.29 U$59.30 U$59.31/A12 U$59.32/A13 U$59.33/A14 U$59.34/A15 U$59.35/A16 U$59.36/A17 U$59.37/A18 U$59.38/A19 U$59.39/A20 U$59.A10 U$59.A11 U$59.A22/DAC1 U$59.AGND U$59.AREF U$59.GND2 U$59.GND3 U$59.PROG U$59.RESET U$59.U5V U$59.UD+ U$59.UD- U$59.UGND1 U$59.UGND2 U$59.VBAT U$59.VUSB

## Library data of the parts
J1 = SparkFun-Connectors:CONN_05X2: Multi connection point. Often used as Generic Header-pin footprint for 0.1 inch spaced/style header connections For AVR SPI programming port, see special device with nice symbol: "AVR_SPI_PROG_5x2.dev" You can populate with any combo of single row headers, but if you'd like an exact match, check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; PROD_ID: CONN-08671; SF_ID: PRT-08506
PAD1-PAD138 = wirepad:1,6/0,8: THROUGH-HOLE PAD
R1-R5 R5V R6-R69 RG = eagle-ltspice:R: RESISTOR, European symbol; SPICEMODEL: NONE; SPICEPREFIX: R
U1-U18 = Texas Instruments_By_element14_Batch_1:TPIC6B595DW: Power Logic 8-Bit Shift Register; MPN: TPIC6B595DW; OC_FARNELL: 1491696; OC_NEWARK: 52F2783; PACKAGE: SOIC-20; SUPPLIER: Texas Instruments
U19 = SparkFun-DigitalIC:TXB0104PWR: 4-Bit Bi-Directional Level Shifter 1.2V-3.6V (VCCA) to 1.65V-5.5V (VCCB) bi-directional level shifter with auto direction sensing. Max data rate - VCCA 1.8V: 20Mbps (50ns), VCCA 3.3V: 100Mbps (10ns) Digikey: 296-21929-1-ND (TSSOP) IC-11329; PROD_ID: IC-11329
U$59 = Teensy356:TEENSY_3.5/3.6

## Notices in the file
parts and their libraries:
SparkFun-DigitalIC: Licensing: Creative Commons ShareAlike 4.0 International - https://creativecommons.org/licenses/by-sa/4.0
